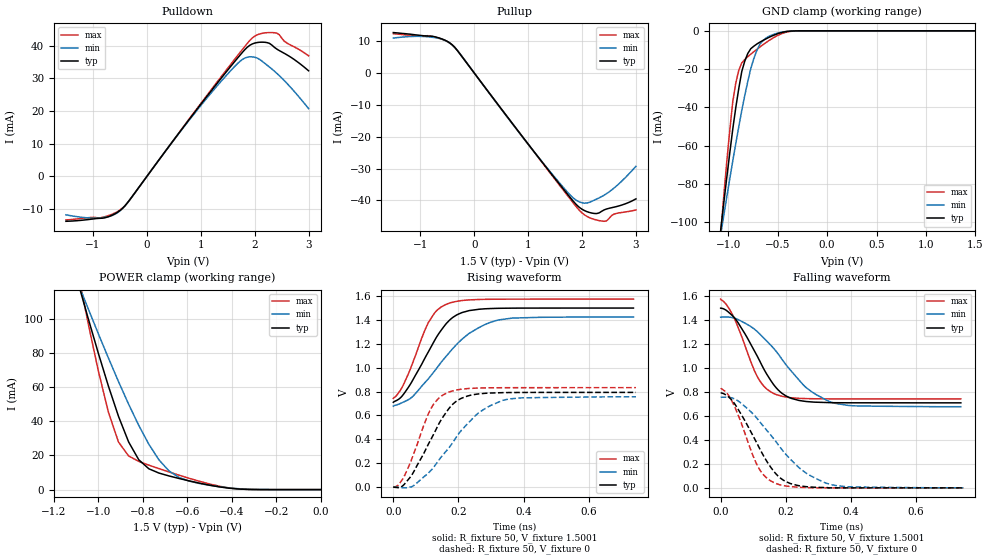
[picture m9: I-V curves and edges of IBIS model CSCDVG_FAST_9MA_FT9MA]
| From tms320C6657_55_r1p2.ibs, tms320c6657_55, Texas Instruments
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|   Model Cell CSCDVG_FAST_9MA_FT9MA
|FAST_9MA
[Model]   CSCDVG_FAST_9MA_FT9MA
Model_type   I/O
Polarity   Non-Inverting
Enable   Active-Low
Cref =  4.0000pF
Rref =  100.0000M
Vref =  0V
Vmeas =  0.75
C_comp   1.5249p   1.4275p   1.6205p
|[mode_tieoffpin] SR1=0  SR0=1 I0=1 I1=0 I2=1
[Model Spec]
Vinl   0.6125   0.6125   0.6125
Vinh   0.9625   0.9625   0.9625
D_overshoot_high 1.95 1.95 1.95
D_overshoot_low -0.3 -0.3 -0.3
D_overshoot_time 1E-9 1E-9 1E-9
S_overshoot_high 1.575 1.575 1.575
S_overshoot_low 0 0 0
[Receiver Thresholds]
Reference_supply Pullup_ref
Threshold_sensitivity= 0.5
Tslew_ac= 5nS
Vinh_ac= +175mV
Vinh_dc= +100mV
Vinl_ac= -175mV
Vinl_dc= -100mV
Vth = 0.75
Vth_max= 0.79
Vth_min= 0.71
[Pullup Reference] 1.5001   1.425   1.575
[Add Submodel]
|Submodel_name Mode
CSCDVG_FT_TH_9MA Non-Driving
[Temperature Range]   25   105   -40
[Voltage Range]   1.5   1.425   1.575
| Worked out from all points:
|   slope of the pulldown table from 0 to 0.225 V, typ, clamps not added: 44.4 ohm
|   slope of the pullup table from 0 to 0.225 V, typ, clamps not added: 44.4 ohm
|   GND clamp passes 1 mA (typ) near -0.47 V on its own axis
|   POWER clamp passes 1 mA (typ) near -0.42 V on its own axis
|   rising waveform, R_fixture 50, V_fixture 1.5001: 20-80 % time 101ps typ, 145ps min, 74.9ps max; typ from 0.71 V to 1.5 V
|   rising waveform, R_fixture 50, V_fixture 0: 20-80 % time 95.7ps typ, 135ps min, 71.1ps max; typ from 0 V to 0.793 V
|   falling waveform, R_fixture 50, V_fixture 1.5001: 20-80 % time 99.3ps typ, 144ps min, 73.9ps max; typ from 1.5 V to 0.709 V
|   falling waveform, R_fixture 50, V_fixture 0: 20-80 % time 99ps typ, 145ps min, 72ps max; typ from 0.792 V to 0 V
[POWER_clamp]
|   voltage   I(typ)   I(min)   I(max)
-1.5V     321.7mA    260.6mA    415.9mA
-1.076V   114.2mA    115.8mA    116.9mA
-1.061V   107.2mA    110.9mA    107.1mA
-954.6mV  60.59mA    77.06mA    45.35mA
-909.2mV  42.85mA    63.21mA    27.81mA
-863.7mV  27.9mA     49.99mA    19.69mA
-818.2mV  17.49mA    37.63mA    16.52mA
-772.8mV  12.19mA    26.53mA    14.33mA
-681.9mV  7.985mA    10.89mA    10.33mA
-590.9mV  5.094mA    4.955mA    6.6mA
-363.7mV  298.5uA    465.2uA    297.6uA
0V        1.518nA    24.08nA    367.8pA
[Pulldown]
|   voltage   I(typ)   I(min)   I(max)
-1.5V     -13.72mA   -11.73mA   -13.31mA
-863.7mV  -12.8mA    -12.65mA   -12.66mA
-500mV    -10.46mA   -10.55mA   -10.29mA
-318.2mV  -7.172mA   -7.186mA   -7.182mA
1.046V    23.05mA    22.61mA    23.31mA
1.591V    34.39mA    33mA       35.06mA
1.818V    38.82mA    36.24mA    39.81mA
1.955V    40.55mA    36.61mA    42.37mA
2.091V    41.08mA    35.83mA    43.61mA
2.273V    40.74mA    33.5mA     44.04mA
2.364V    39.55mA    32.26mA    43.99mA
3V        32.34mA    20.77mA    36.92mA
[Pullup]
|   voltage   I(typ)   I(min)   I(max)
-1.5V     12.66mA    10.94mA    12.31mA
-818.2mV  11.55mA    11.26mA    11.58mA
-590.9mV  10.61mA    10.52mA    10.54mA
-409.1mV  8.836mA    8.777mA    8.84mA
1.227V    -27.25mA   -27.19mA   -27.38mA
1.727V    -37.96mA   -37.32mA   -38.38mA
1.909V    -41.55mA   -40.1mA    -42.29mA
2.046V    -43.18mA   -40.84mA   -44.51mA
2.227V    -44.08mA   -39.9mA    -45.94mA
2.409V    -42.96mA   -38.35mA   -46.53mA
2.591V    -42.11mA   -36.14mA   -44.31mA
3V        -39.5mA    -29.28mA   -42.98mA
[GND_clamp]
|   voltage   I(typ)   I(min)   I(max)
-1.5V     -310.1mA   -250.5mA   -402.5mA
-1.076V   -103.6mA   -106.2mA   -105.2mA
-1.046V   -89.81mA   -96.36mA   -86.02mA
-954.6mV  -51.22mA   -67.87mA   -36.88mA
-924.3mV  -40.08mA   -58.86mA   -27.29mA
-863.7mV  -21.24mA   -41.56mA   -16.73mA
-833.4mV  -15.8mA    -33.75mA   -15.03mA
-772.8mV  -9.345mA   -19.75mA   -12.19mA
-712.2mV  -6.928mA   -10.35mA   -9.704mA
-621.3mV  -4.261mA   -3.896mA   -6.225mA
-409.1mV  -337.1uA   -289.1uA   -618.9uA
1.5V      1.518nA    257.2nA    299pA
[Ramp]
| variable   typ   min   max
dV/dt_f   0.632752/0.14700507n   0.598864/0.21860086n   0.666584/0.11454368n
dV/dt_r 0.63894896/0.14120975n 0.61111208/0.20900305n 0.66816984/0.10960734n
R_load = 50
[Rising Waveform]
R_fixture = 50
V_fixture = 1.5001
V_fixture_min = 1.425
V_fixture_max = 1.575
|   time   V(typ)   V(min)   V(max)
0s        709.9mV    677.4mV    742.6mV
33.32ps   784.9mV    714.7mV    870.8mV
61.63ps   905.8mV    764.2mV    1.056V
107.8ps   1.134V     907.4mV    1.38V
130.6ps   1.247V     986.7mV    1.471V
163.8ps   1.374V     1.101V     1.533V
196ps     1.445V     1.2V       1.557V
233.2ps   1.479V     1.289V     1.569V
325.6ps   1.498V     1.402V     1.574V
737.1ps   1.5V       1.425V     1.575V
[Rising Waveform]
R_fixture = 50
V_fixture = 0
V_fixture_min = 0
V_fixture_max = 0
|   time   V(typ)   V(min)   V(max)
0s        0V         0V         0V
14.24ps   -5.641mV   -1.838mV   12.44mV
34.98ps   26.64mV    -7.269mV   97.78mV
61.77ps   123.4mV    10.36mV    272.8mV
118.7ps   415.6mV    147.9mV    673mV
170.6ps   657.5mV    327.9mV    795.5mV
206.5ps   740.4mV    467mV      818.8mV
257.6ps   778.8mV    612mV      829mV
336.3ps   790.9mV    726.9mV    832.1mV
744.7ps   793mV      756.2mV    832.8mV
[Falling Waveform]
R_fixture = 50
V_fixture = 1.5001
V_fixture_min = 1.425
V_fixture_max = 1.575
|   time   V(typ)   V(min)   V(max)
0s        1.499V     1.424V     1.575V
38.29ps   1.431V     1.419V     1.433V
115.2ps   1.083V     1.296V     914.4mV
139.3ps   958.4mV    1.23V      830.2mV
165.9ps   849.6mV    1.154V     783.8mV
201.5ps   765.5mV    1.023V     757.6mV
258.6ps   722mV      845.9mV    744.9mV
339ps     710.9mV    714.3mV    742.4mV
408.7ps   709.6mV    684.2mV    742.1mV
737.1ps   709.3mV    676.9mV    741.9mV
[Falling Waveform]
R_fixture = 50
V_fixture = 0
V_fixture_min = 0
V_fixture_max = 0
|   time   V(typ)   V(min)   V(max)
0s        792.3mV    755.5mV    831.9mV
19.58ps   768.6mV    756mV      789.2mV
40.67ps   709.7mV    744.7mV    690.6mV
114ps     357.4mV    571.7mV    179mV
139.3ps   231.8mV    487.4mV    86.92mV
169.1ps   118.3mV    387.1mV    36.92mV
197.8ps   55.44mV    286.1mV    16.35mV
247.4ps   14.86mV    152.6mV    4.302mV
340.9ps   0V         26.03mV    0V
744.7ps   0V         0V         0V
